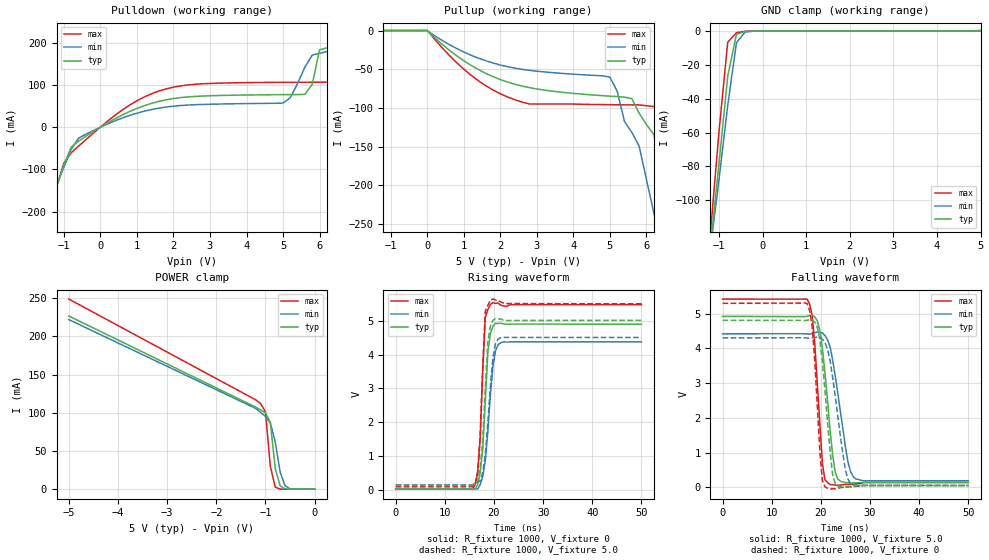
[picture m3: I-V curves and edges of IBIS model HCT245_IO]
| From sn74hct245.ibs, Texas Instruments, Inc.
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|   Model HCT245_IO
[Model]   HCT245_IO
Model_type  I/O
Polarity   Non-Inverting
Enable   Active-Low
Vmeas = 1.3v
Cref = 50pf
Rref = 1000
Vinl = 0.8
Vinh = 2.0
| variable   typ   min   max
C_comp   4.0pF   NA   NA
[Temperature Range]   25   85   -40
[Voltage Range]   5.0   4.5   5.5
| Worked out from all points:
|   slope of the pulldown table from 0 to 0.75 V, typ, clamps not added: 21.5 ohm
|   slope of the pullup table from 0 to 0.75 V, typ, clamps not added: 24.7 ohm
|   GND clamp passes 1 mA (typ) near -0.50 V on its own axis
|   POWER clamp passes 1 mA (typ) near -0.62 V on its own axis
|   rising waveform, R_fixture 1000, V_fixture 0: 20-80 % time 1.14ns typ, 1.45ns min, 1.01ns max; typ from 0.013 V to 4.9 V
|   falling waveform, R_fixture 1000, V_fixture 5.0: 20-80 % time 1.94ns typ, 2.65ns min, 1.47ns max; typ from 4.92 V to 0.142 V
|   rising waveform, R_fixture 1000, V_fixture 5.0: 20-80 % time 1.14ns typ, 1.4ns min, 984ps max; typ from 0.124 V to 5.02 V
|   falling waveform, R_fixture 1000, V_fixture 0: 20-80 % time 1.79ns typ, 2.46ns min, 1.33ns max; typ from 4.81 V to 0.048 V
[Pulldown]
|   Voltage   I(typ)   I(min)   I(max)
-5V       -1.022A    -961.6mA   -1.156A
-1.6V     -226.3mA   -218.2mA   -231.2mA
-1V       -89.9mA    -95.21mA   -85.71mA
-600mV    -33.15mA   -26.42mA   -45.31mA
1.6V      61.02mA    45.03mA    85.51mA
5V        77.01mA    57.19mA    106.2mA
5.6V      77.67mA    142.5mA    106.3mA
5.8V      101.5mA    170.8mA    106.4mA
6V        183.3mA    174.9mA    106.4mA
6.4V      192.6mA    183.2mA    110.5mA
6.6V      197.3mA    187.3mA    212.5mA
10V       274.3mA    256.7mA    305mA
[Pullup]
|   Voltage   II(typ)   I(min)   I(max)
-5V       43.13uA    102.7uA    672.6uA
0V        43.13uA    102.7uA    672.6uA
1.2V      -44.73mA   -31.58mA   -57.47mA
2.2V      -66.34mA   -46.43mA   -85.65mA
5V        -84.57mA   -59.91mA   -95.63mA
5.6V      -87.77mA   -131.4mA   -95.84mA
5.8V      -106.5mA   -149.2mA   -95.91mA
6.2V      -134.2mA   -234.9mA   -97.97mA
6.4V      -173.1mA   -276.4mA   -107mA
6.8V      -269.1mA   -370.1mA   -145mA
7.2V      -378.9mA   -463.7mA   -255.8mA
10V       -1.142A    -1.12A     -1.083A
[GND Clamp]
|   Voltage   I(typ)   I(min)   I(max)
-5V       -1.077A    -924.7mA   -1.269A
-1.2V     -128.1mA   -129.6mA   -120.4mA
-1V       -78.37mA   -87.72mA   -59.37mA
-800mV    -26.64mA   -43.97mA   -6.54mA
-600mV    -1.813mA   -6.845mA   -911.6uA
-400mV    -164.5uA   -447.9uA   -20.92uA
-200mV    -653.3nA   -11.11uA   -1.337uA
4.8V      465.5pA    2.542uA    13.12uA
5V        465.5pA    526.2uA    13.79uA
[POWER Clamp]
|   Voltage   I(typ)   I(min)   I(max)
-5V       226.8mA    222.1mA    249mA
-1.2V     107.5mA    105.8mA    117.1mA
-1.1V     103.8mA    100.6mA    112.4mA
-1V       100mA      95.3mA     101.3mA
-900mV    87.37mA    86.47mA    29.69mA
-800mV    26.85mA    61.94mA    2.641mA
-700mV    4.174mA    22.04mA    174.9uA
-600mV    355.3uA    4.483mA    22.11uA
-500mV    20.77uA    526.2uA    17.2uA
40.86fV   430.9pA    32.45nA    154.9nA
[Ramp]
| variable   typ   min   max
dV/dt_r  2.874E+00/9.880E-10  2.580E+00/1.319E-09  3.162E+00/8.060E-10
dV/dt_f  2.904E+00/1.785E-09  2.598E+00/2.509E-09  3.186E+00/1.329E-09
R_load = 1000
[Rising Waveform]
R_fixture = 1000
V_fixture = 0
V_fixture_min = 0
V_fixture_max = 0
C_fixture = 0pf
L_fixture = 0nH
|   Time   V(typ)   V(min)   V(max)
0s        13.36mV    17mV       12.21mV
16.15ns   13.81mV    16.52mV    147.1mV
16.67ns   147.2mV    16.64mV    475.8mV
17.19ns   495.8mV    147.1mV    1.5V
18.23ns   2.594V     857.6mV    5.1V
18.75ns   4.08V      1.721V     5.338V
19.27ns   4.633V     2.819V     5.492V
20.31ns   4.931V     4.114V     5.522V
21.88ns   4.914V     4.379V     5.448V
50ns      4.904V     4.379V     5.483V
[Falling Waveform]
R_fixture = 1000
V_fixture = 5.0
V_fixture_min = 4.5
V_fixture_max = 5.5
C_fixture = 0pf
L_fixture = 0nH
|   Time   V(typ)   V(min)   V(max)
0s        4.919V     4.418V     5.416V
17.19ns   4.918V     4.415V     5.416V
18.23ns   4.949V     4.426V     4.95V
19.79ns   4.524V     4.463V     1.836V
20.31ns   3.996V     4.443V     687.3mV
21.35ns   2.501V     4.252V     137.9mV
22.92ns   438.8mV    3.209V     66.68mV
25.52ns   131.4mV    722.7mV    85.15mV
26.56ns   132.1mV    312mV      91.1mV
50ns      141.8mV    190.7mV    140.2mV
[Rising Waveform]
R_fixture = 1000
V_fixture = 5.0
V_fixture_min = 4.5
V_fixture_max = 5.5
C_fixture = 0pf
L_fixture = 0nH
|   Time   V(typ)   V(min)   V(max)
0s        123.5mV    141.7mV    84.1mV
16.15ns   177.9mV    183.4mV    144.2mV
17.19ns   636.1mV    259.9mV    1.634V
17.71ns   1.469V     514.1mV    3.664V
18.23ns   3.027V     1.034V     5.292V
18.75ns   4.375V     2.002V     5.465V
19.27ns   4.852V     3.086V     5.619V
20.31ns   5.067V     4.327V     5.62V
21.35ns   5.057V     4.504V     5.561V
50ns      5.02V      4.51V      5.509V
[Falling Waveform]
R_fixture = 1000
V_fixture = 0
V_fixture_min = 0
V_fixture_max = 0
C_fixture = 0pf
L_fixture = 0nH
|   Time   V(typ)   V(min)   V(max)
0s        4.806V     4.3V       5.295V
17.19ns   4.806V     4.296V     5.29V
18.23ns   4.815V     4.301V     4.635V
19.27ns   4.602V     4.322V     2.359V
20.31ns   3.612V     4.265V     195.3mV
20.83ns   2.792V     4.166V     15.41mV
22.4ns    348.8mV    3.16V      -36.01mV
25ns      18.31mV    493.8mV    8.24mV
26.04ns   28.38mV    111.4mV    16.33mV
50ns      48.04mV    55.72mV    55.05mV
